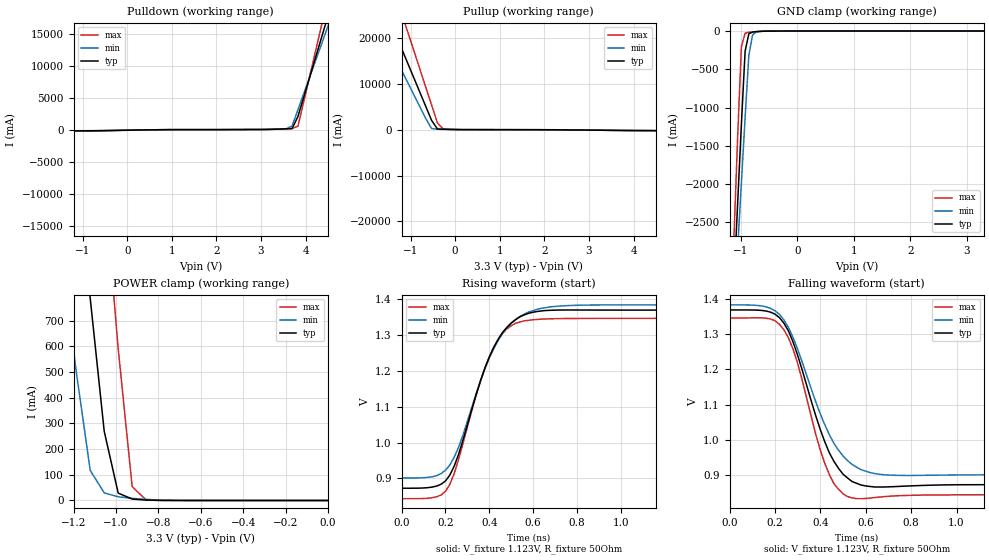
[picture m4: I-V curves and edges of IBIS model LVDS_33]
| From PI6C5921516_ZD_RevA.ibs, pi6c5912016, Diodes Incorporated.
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|   Model OUTPUT  LVDS_33
[Model]  LVDS_33
Model_type  3-state
Vmeas =   1.65V
|Variable   typ   min   max
C_comp   2.100p   2.042p   2.118p
[Voltage Range]   3.300V   3.135V   3.465V
[GND Clamp Reference]   0.000V   0.000V   0.000V
[POWER Clamp Reference]   3.300V   3.135V   3.465V
[Pullup Reference]   3.300V   3.135V   3.465V
[Pulldown Reference]   0.000V   0.000V   0.000V
[Temperature Range]   25   85   -40
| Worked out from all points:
|   slope of the pulldown table from 0 to 0.495 V, typ, clamps not added: 8.87 ohm
|   slope of the pullup table from 0 to 0.495 V, typ, clamps not added: 22.3 ohm
|   GND clamp passes 1 mA (typ) near -0.53 V on its own axis
|   POWER clamp passes 1 mA (typ) near -0.83 V on its own axis
|   falling waveform, V_fixture 1.123V, R_fixture 50Ohm: 20-80 % time 150ps typ, 171ps min, 128ps max; typ from 1.37 V to 0.873 V
|   rising waveform, V_fixture 1.123V, R_fixture 50Ohm: 20-80 % time 162ps typ, 177ps min, 150ps max; typ from 0.873 V to 1.37 V
[GND Clamp]
| Voltage   I(typ)   I(min)   I(max)
-3.3V     -37.33A    -32.1A     -46.15A
-1.122V   -3.273A    -3.698A    -2.691A
-1.056V   -2.245A    -2.84A     -1.378A
-990mV    -1.217A    -1.983A    -203.1mA
-924mV    -263.1mA   -1.127A    -28.5mA
-858mV    -35.97mA   -315.8mA   -16.19mA
-792mV    -13.16mA   -50.06mA   -11.43mA
-726mV    -7.743mA   -13.4mA    -7.263mA
-528mV    -940.7uA   -1.475mA   -418.2uA
3.3V      22.11uA    30.12uA    13.6uA
[POWER Clamp]
| Voltage   I(typ)   I(min)   I(max)
-3.3V     23.39A     18.39A     31.56A
-1.254V   1.821A     934.2mA    3.226A
-1.188V   1.303A     501.5mA    2.566A
-1.122V   786.1mA    117mA      1.907A
-1.056V   269.6mA    29.68mA    1.248A
-990mV    28.82mA    14.37mA    590.6mA
-924mV    5.681mA    8.377mA    53.86mA
-858mV    1.601mA    4.452mA    2.177mA
-660mV    59.08uA    190.2uA    52.67uA
0V        22.11uA    22.52uA    21.08uA
[Pulldown]
| Voltage   I(typ)   I(min)   I(max)
-3.3V     -64.21A    -57.12A    -76.47A
-2.244V   -17.37A    -15.88A    -20A
-2.112V   -14.3A     -13.33A    -16.07A
-1.584V   -2.039A    -3.124A    -502mA
-1.452V   -203.2mA   -592.9mA   -231.5mA
-1.32V    -188.9mA   -165mA     -223.9mA
3.036V    30.85mA    39.51mA    35.7mA
3.696V    177.9mA    578.8mA    170.3mA
3.828V    2.064A     3.117A     551.9mA
4.356V    14.37A     13.35A     16.25A
4.488V    17.45A     15.91A     20.19A
6.6V      129.7A     111.5A     160.5A
[Pullup]   |Note: Vtable = Vcc - Voutput
| Voltage   I(typ)   I(min)   I(max)
-3.3V     129.7A     103A       173.6A
-1.716V   31.65A     22.99A     48.16A
-1.452V   23.57A     17.81A     32.95A
-1.188V   17.43A     12.7A      25.08A
-1.056V   14.36A     10.14A     21.15A
-528mV    2.042A     255.1mA    5.391A
-264mV    100.9mA    79.68mA    140.6mA
4.488V    -198mA     -178.9mA   -228.2mA
4.752V    -211.2mA   -3.761A    -235.8mA
5.016V    -5.099A    -8.863A    -269.2mA
5.808V    -23.49A    -24.83A    -22.94A
6.6V      -64.2A     -65.62A    -63.38A
[Falling Waveform]
V_fixture = 1.123V
V_fixture_min = 1.145V
V_fixture_max = 1.10V
R_fixture = 50Ohm
C_fixture = 0F
|   Time   V(typ)   V(min)   V(max)
0s        1.369V     1.384V     1.347V
160ps     1.367V     1.379V     1.346V
240ps     1.331V     1.341V     1.312V
300ps     1.241V     1.258V     1.218V
380ps     1.068V     1.108V     1.015V
420ps     993.6mV    1.042V     932.2mV
480ps     918.7mV    970.5mV    858.8mV
540ps     881mV      929.8mV    834.6mV
740ps     867mV      898.6mV    840.6mV
4ns       872.7mV    901.2mV    843.4mV
[Rising Waveform]
V_fixture = 1.123V
V_fixture_min = 1.145V
V_fixture_max = 1.10V
R_fixture = 50Ohm
C_fixture = 0F
|   Time   V(typ)   V(min)   V(max)
0s        872.7mV    901.2mV    843.4mV
140ps     875.9mV    904.6mV    846.3mV
200ps     892.8mV    923mV      864.1mV
260ps     967.4mV    987mV      953.2mV
360ps     1.173V     1.173V     1.172V
420ps     1.265V     1.262V     1.266V
480ps     1.321V     1.319V     1.317V
560ps     1.357V     1.359V     1.34V
860ps     1.37V      1.384V     1.347V
4ns       1.369V     1.384V     1.347V
[Ramp]
|   typ   min   max
dV/dt_r   0.5004V/222.86p   0.474V/208.90p   0.5173V/230.54p
dV/dt_f   0.5004V/141.87p   0.474V/150.99p   0.5173V/114.18p
R_load =   50.0000
